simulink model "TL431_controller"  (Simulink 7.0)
settings: Solver=ode23tb  SolverMode=SingleTasking  StartTime=0.0  StopTime=100e-3  RelTol=1e-6
undefined symbols (not defined in the file or in its folder): plecs

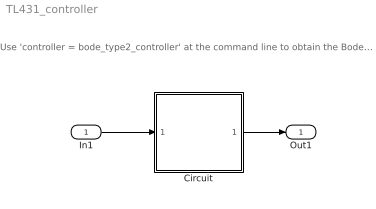
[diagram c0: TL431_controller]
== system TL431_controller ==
  note: Use 'controller = bode_type2_controller' at the command line to obtain the Bode plot
  In1 : Inport  OutDataType=sfix(16)  OutScaling=2^0
  Circuit : Subsystem  LoadFcn=plecs('sl', 200);  InitFcn=plecs('sl', 214);  StartFcn=plecs('sl', 208);  StopFcn=plecs('sl', 209);  mask(PlecsCircuit){PLECSData=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}
      mask prompts: PLECSData "PLECS Data (Do not delete or modify!)"
      mask init:
      | % PLACE CUSTOM INITIALIZATIONS ABOVE
      | % DO NOT REMOVE
      | plecs('sl', 215);
      | % DO NOT REMOVE
  Out1 : Outport  OutDataType=sfix(16)  OutScaling=2^0
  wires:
  In1/1 -> Circuit/1(In1)
  Circuit/1(Out1) -> Out1/1

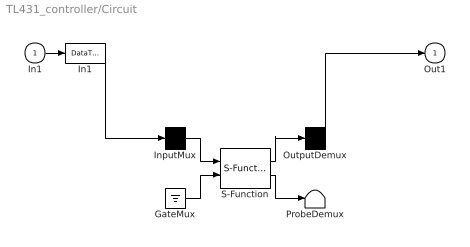
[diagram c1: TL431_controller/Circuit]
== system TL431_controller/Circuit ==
  In1 : Inport  PortDimensions=1
  " GateMux " : Ground
  " In1 " : DataTypeConversion
  " InputMux " : Mux  Inputs=[ 1 ]
  " OutputDemux " : Demux  Outputs=[ 1 ]
  " ProbeDemux " : Terminator
  " S-Function " : S-Function  FunctionName=plecs
  Out1 : Outport  PortDimensions=1
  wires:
  " S-Function "/1 -> " OutputDemux "/1
  " InputMux "/1 -> " S-Function "/1
  " GateMux "/1 -> " S-Function "/2
  " S-Function "/2 -> " ProbeDemux "/1
  In1/1 -> " In1 "/1
  " In1 "/1 -> " InputMux "/1
  " OutputDemux "/1 -> Out1/1
